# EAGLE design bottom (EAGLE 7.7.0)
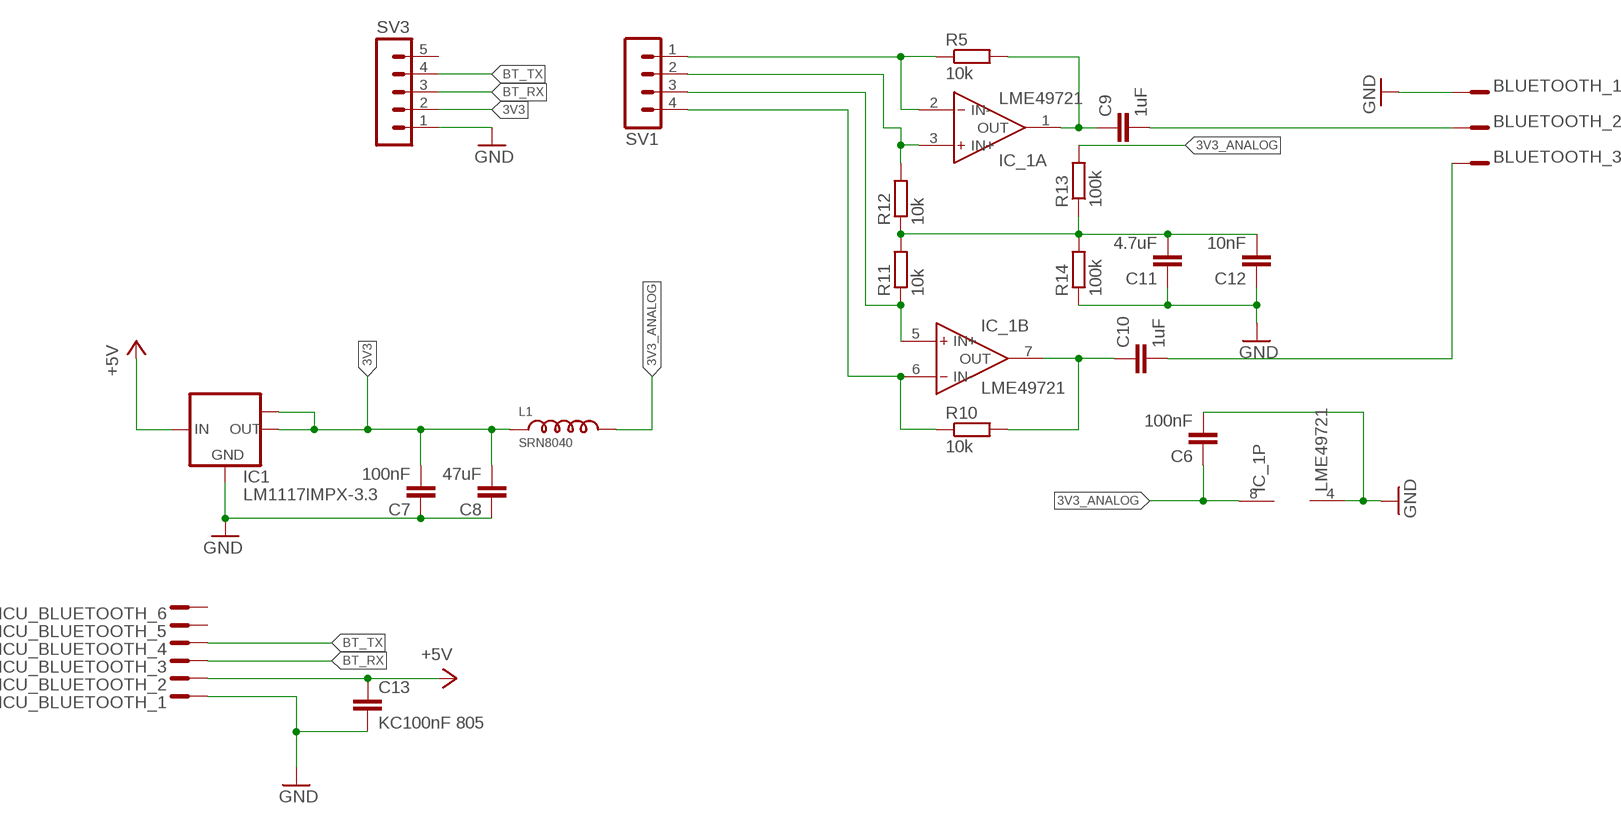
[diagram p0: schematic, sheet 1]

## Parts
BLUETOOTH  JST_3_PIN_B3B-PH-KS  [B3B-PH-KS]
C6  100nF  C-EUC0805  [C0805]
C7  100nF  C-EUC0805  [C0805]
C8  47uF  C-EUC0805K  [C0805K]
C9  1uF  C-EUC0805  [C0805]
C10  1uF  C-EUC0805  [C0805]
C11  4.7uF  C-EUC0805  [C0805]
C12  10nF  C-EUC0805  [C0805]
C13  KC100nF 805  C-EUC0805  [C0805]
IC1  LM1117IMPX-3.3  [SOT223]
IC_1  LME49721  LME49721LME49721  [SOIC-8_NARROW]
L1  SRN8040  [INDUCTOR_8X8]
MCU_BLUETOOTH  JST_6_PIN_B6B-PH-KS  [B6B-PH-KS]
R5  10k  R-EU_R0805  [R0805]
R10  10k  R-EU_R0805  [R0805]
R11  10k  R-EU_R0805  [R0805]
R12  10k  R-EU_R0805  [R0805]
R13  100k  R-EU_R0805  [R0805]
R14  100k  R-EU_R0805  [R0805]
SV1  MA04-1  [MA04-1]
SV3  MA05-1  [MA05-1]

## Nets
3V3: C7.2 C8.2 IC1.2(OUT) IC1.TAB(OUT1) L1.P$1 SV3.2
3V3_ANALOG: C6.1 IC_1.8(P:V+) L1.P$2 R13.2
+5V: C13.1 IC1.3(IN) MCU_BLUETOOTH.P$2
BT_AUDIO_L_OUT: BLUETOOTH.P$2 C9.2
BT_AUDIO_R_OUT: BLUETOOTH.P$3 C10.2
BT_RX: MCU_BLUETOOTH.P$3 SV3.3
BT_TX: MCU_BLUETOOTH.P$4 SV3.4
GND: BLUETOOTH.P$1 C6.2 C7.1 C8.1 C11.1 C12.1 C13.2 IC1.1(GND) IC_1.4(P:V-) MCU_BLUETOOTH.P$1 R14.1 SV3.1
N$7: IC_1.2(A:IN-) R5.1 SV1.1
N$10: IC_1.3(A:IN+) R12.2 SV1.2
N$12: IC_1.5(B:IN+) R11.1 SV1.3
N$13: IC_1.6(B:IN-) R10.1 SV1.4
N$20: C9.1 IC_1.1(A:OUT) R5.2
N$21: C10.1 IC_1.7(B:OUT) R10.2
N$23: C11.2 C12.2 R11.2 R12.1 R13.1 R14.2
Unconnected: MCU_BLUETOOTH.P$5 MCU_BLUETOOTH.P$6 SV3.5

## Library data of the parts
BLUETOOTH = conn-JST:JST_3_PIN_
C6-C13 = rcl:C-EU: CAPACITOR, European symbol
IC1 = lm1117:LM1117IMPX-*
IC_1 = lme49721:LME49721
L1 = ferrit_bear:SRN8040
MCU_BLUETOOTH = conn-JST:JST_6_PIN_
R5 R10-R14 = resistor:R-EU_: RESISTOR, European symbol
SV1 = con-lstb:MA04-1: PIN HEADER; OC_FARNELL: unknown; OC_NEWARK: unknown
SV3 = con-lstb:MA05-1: PIN HEADER; OC_FARNELL: unknown; OC_NEWARK: unknown

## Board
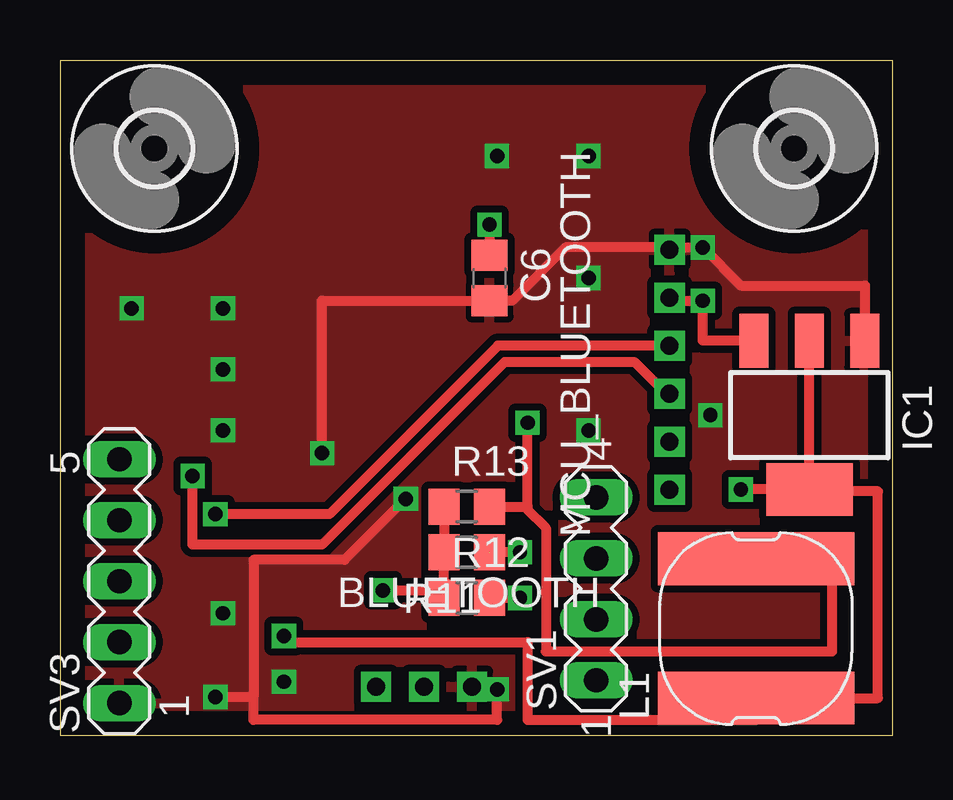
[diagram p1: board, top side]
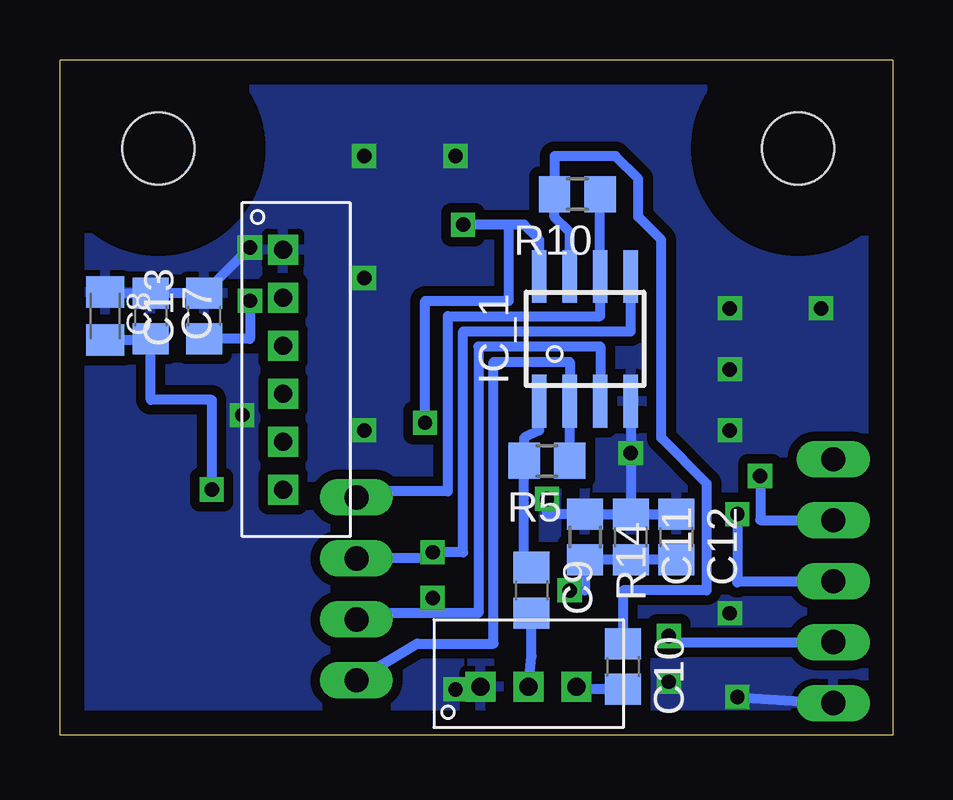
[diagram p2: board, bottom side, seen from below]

Size 34.71 x 28.13 mm. Coordinates in mm from the lower left corner, seen from the top.
Outline: 0,0 34.71,0 34.71,28.13 0,28.13 0,0
Copper layers (1*16): Top 0.035mm / dielectric 1.5mm / Bottom 0.035mm
Design rules "default": minimum track width 10mil, minimum drill 24mil, track to track 8mil, track to pad 8mil, pad to pad 8mil, via to via 8mil, smd to smd 8mil, copper to edge 40mil, drill to drill 8mil, minimum pad ring 10mil, minimum via ring 8mil, stop-mask expansion 4mil, vias tented up to drill 0mil, thermal gap 10mil

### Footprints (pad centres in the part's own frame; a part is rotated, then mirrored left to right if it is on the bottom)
B3B-PH-KS = drill 0.75 pad 1.2 square: P$1 -2,1.7; P$2 -4,1.7; P$3 -6,1.7
C0805 = smd 1.3 x 1.5: 1 -0.95,0; 2 0.95,0
C0805K = smd 1.3 x 1.6: 1 -1,0; 2 1,0
SOT223 = smd 1.219 x 2.235: 1 -2.311,-3.099; 2 0,-3.099; 3 2.311,-3.099 | smd 3.6 x 2.2: TAB 0,3.099
SOIC-8_NARROW = smd 0.6 x 2.2: 1 -1.905,-2.6; 2 -0.635,-2.6; 3 0.635,-2.6; 4 1.905,-2.6; 5 1.905,2.6; 6 0.635,2.6; 7 -0.635,2.6; 8 -1.905,2.6
INDUCTOR_8X8 = smd 2.2 x 8.2: P$1 -2.9,0; P$2 2.9,0
B6B-PH-KS = drill 0.75 pad 1.2 square: P$1 -2,1.7; P$2 -4,1.7; P$3 -6,1.7; P$4 -8,1.7; P$5 -10,1.7; P$6 -12,1.7
R0805 = smd 1.3 x 1.5: 1 -0.95,0; 2 0.95,0
MA04-1 = drill 1.016 long: 1 -3.81,0; 2 -1.27,0; 3 1.27,0; 4 3.81,0
MA05-1 = drill 1.016 long: 1 -5.08,0; 2 -2.54,0; 3 0,0; 4 2.54,0; 5 5.08,0
3,0 = hole 3: 0,0

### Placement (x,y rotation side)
BLUETOOTH  19.18,0.32 0 top
C6  17.91,19.05 270 top
C7  30.92,17.46 270 bottom
C8  32.83,17.46 270 bottom
C9  15.05,6.03 270 bottom
C10  11.24,2.86 270 bottom
C11  10.92,8.25 270 bottom
C12  9.02,8.25 270 bottom
C13  28.7,17.46 90 bottom
IC1  31.24,13.33 180 top
IC_1  12.83,16.51 0 bottom
L1  29.02,4.44 90 top
MCU_BLUETOOTH  27.11,22.22 90 top
R5  14.41,11.43 180 bottom
R10  13.14,22.54 180 bottom
R11  16.95,7.62 180 top
R12  16.95,5.71 0 top
R13  16.95,9.52 0 top
R14  12.83,8.25 270 bottom
SV1  22.35,6.1 90 top
SV3  2.48,6.41 90 top
U$2  [3,0]  3.94,24.45 0 top
U$3  [3,0]  30.61,24.45 0 top

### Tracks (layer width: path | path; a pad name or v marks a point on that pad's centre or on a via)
3V3  (via drill 0.6)
  Top 0.406: IC1.TAB IC1.2 | L1.P$1 34.1,1.54 34.1,10.16 31.24,10.16 IC1.TAB | IC1.TAB v28.38,10.24 28.38,10.16 | v9.33,4.13 9.33,3.87 19.49,3.87 19.49,0.63 29.02,0.63 L1.P$1 | 29.02,1.59 L1.P$1
  Bottom 0.406: v28.38,10.24 28.38,13.97 30.92,13.97 C7.2 30.92,16.46 C8.2 | v9.33,4.13 9.33,3.87 SV3.2
3V3_ANALOG  (via drill 0.6)
  Top 0.406: v17.91,21.27 C6.1 | 26.75,7.34 L1.P$2 31.88,7.34 31.88,7.3 32.19,7.3 32.19,3.49 20.26,3.49 20.26,8.64 19.49,9.4 19.49,9.52 | R13.2 19.49,9.52 | 19.49,9.52 v19.49,13.02
  Bottom 0.406: IC_1.8 14.73,20.64 15.37,21.27 16,21.27 | 16,21.27 v17.91,21.27 | v19.49,13.02 19.49,18.1 16,18.1 16,21.27
+5V  (via drill 0.6)
  Top 0.406: IC1.3 26.8,16.43 v26.8,18.1 25.41,18.1 MCU_BLUETOOTH.P$2
  Bottom 0.406: v26.8,18.1 26.8,16.51 C13.1
BT_AUDIO_L_OUT
  Bottom 0.406: BLUETOOTH.P$2 15.05,3.29 C9.2
BT_AUDIO_R_OUT
  Bottom 0.406: C10.2 12.86,1.91 BLUETOOTH.P$3
BT_RX  (via drill 0.6)
  Top 0.406: MCU_BLUETOOTH.P$3 18.26,16.22 11.24,9.21 v6.48,9.21
  Bottom 0.406: v6.48,9.21 6.48,6.41 | 6.48,6.35 6.48,6.41 | 6.48,6.41 SV3.3
BT_TX  (via drill 0.6)
  Top 0.406: v5.52,10.79 5.52,7.94 10.92,7.94 18.54,15.56 23.94,15.56 25.27,14.22 MCU_BLUETOOTH.P$4
  Bottom 0.406: v5.52,10.79 5.52,8.95 SV3.4
GND  (via drill 0.6)
  Top 0.406: IC1.1 33.55,18.73 28.38,18.73 v26.8,20.32 25.41,20.32 MCU_BLUETOOTH.P$1 25.32,20.32 21.08,20.32 18.86,18.1 C6.2 10.92,18.1 v10.92,11.75 | v14.41,9.84 11.87,7.3 8.06,7.3 8.06,1.59 | 8.06,1.59 v6.48,1.59 | 8.06,1.59 8.06,0.63 18.22,0.63 v18.22,1.9
  Bottom 0.406: v26.8,20.32 C13.2 C7.1 33.15,18.41 C8.1 | IC_1.4 v10.92,11.75 C11.1 | C11.1 R14.1 14.41,9.21 v14.41,9.84 | C11.1 C12.1 | v6.48,1.59 SV3.1 | v18.22,1.9 18.13,1.9 BLUETOOTH.P$1
  other vias: 6.79,17.78 18.22,24.13 22.03,24.13 22.03,19.05 22.03,12.7 6.79,15.24 6.79,12.7 9.33,2.22 27.11,13.33 6.79,5.08 2.98,17.78
  pour Bottom (isolate 0.406): -0.83,-1.27 -0.83,27.94 39.81,27.94 39.81,-1.27
  pour Top (isolate 0.305): -0.83,27.94 37.27,27.94 37.27,-1.27 -0.83,-1.27
N$7
  Bottom 0.406: R5.1 IC_1.2 | IC_1.2 | IC_1.2 13.46,15.56 16.64,15.56 16.64,3.81 19.81,3.81 SV1.1
N$10  (via drill 0.6)
  Top 0.406: R12.2 v19.18,5.71
  Bottom 0.406: IC_1.3 12.19,16.19 17.27,16.19 17.27,5.08 19.49,5.08 | 19.49,5.08 22.35,5.08 SV1.2 | v19.18,5.71 19.49,5.71 19.49,5.08
N$12  (via drill 0.6)  (1 unrouted)
  Top 0.406: v19.18,7.62 18.22,7.62
  Bottom 0.406: IC_1.5 10.92,16.83 17.91,16.83 R11.1 v19.18,7.62 19.18,7.37 SV1.3
N$13
  Bottom 0.406: R10.1 IC_1.6 12.19,17.46 18.54,17.46 18.54,10.16 22.35,10.16 SV1.4
N$20
  Bottom 0.406: IC_1.1 14.73,12.7 15.36,12.38 R5.2 15.36,7.3 C9.1
N$21
  Bottom 0.406: IC_1.7 13.46,20.96 14.09,21.59 R10.2 14.09,24.13 11.56,24.13 10.6,23.18 10.6,21.59 9.65,20.64 9.65,12.38 7.75,10.48 7.75,6.03 11.24,6.03 C10.1
N$23  (via drill 0.6)
  Top 0.406: R13.1 R11.2 16,6.03 | R12.1 16,6.03 | v13.46,6.03 16,6.03
  Bottom 0.406: C12.2 C11.2 R14.2 12.83,6.03 v13.46,6.03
